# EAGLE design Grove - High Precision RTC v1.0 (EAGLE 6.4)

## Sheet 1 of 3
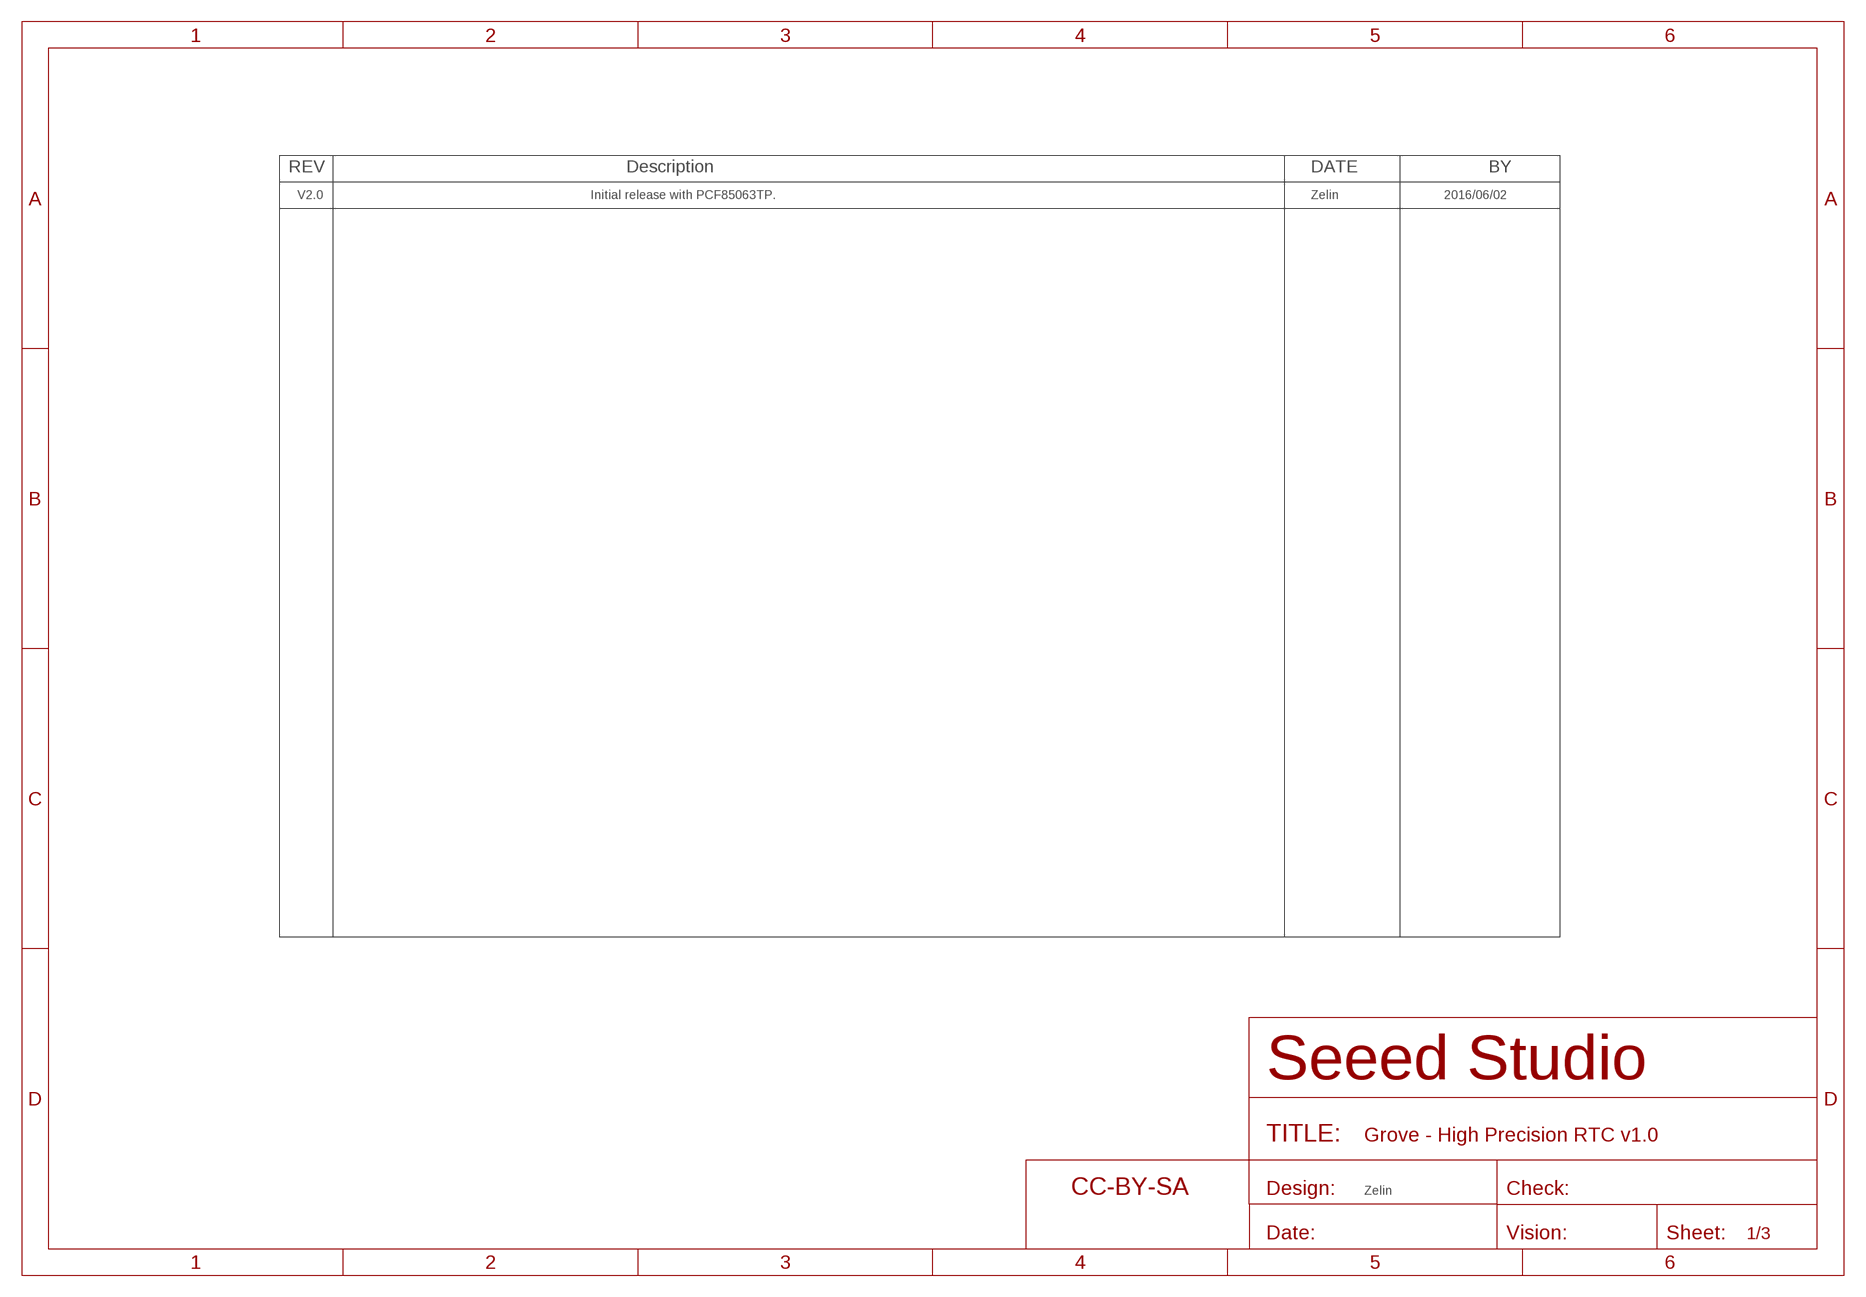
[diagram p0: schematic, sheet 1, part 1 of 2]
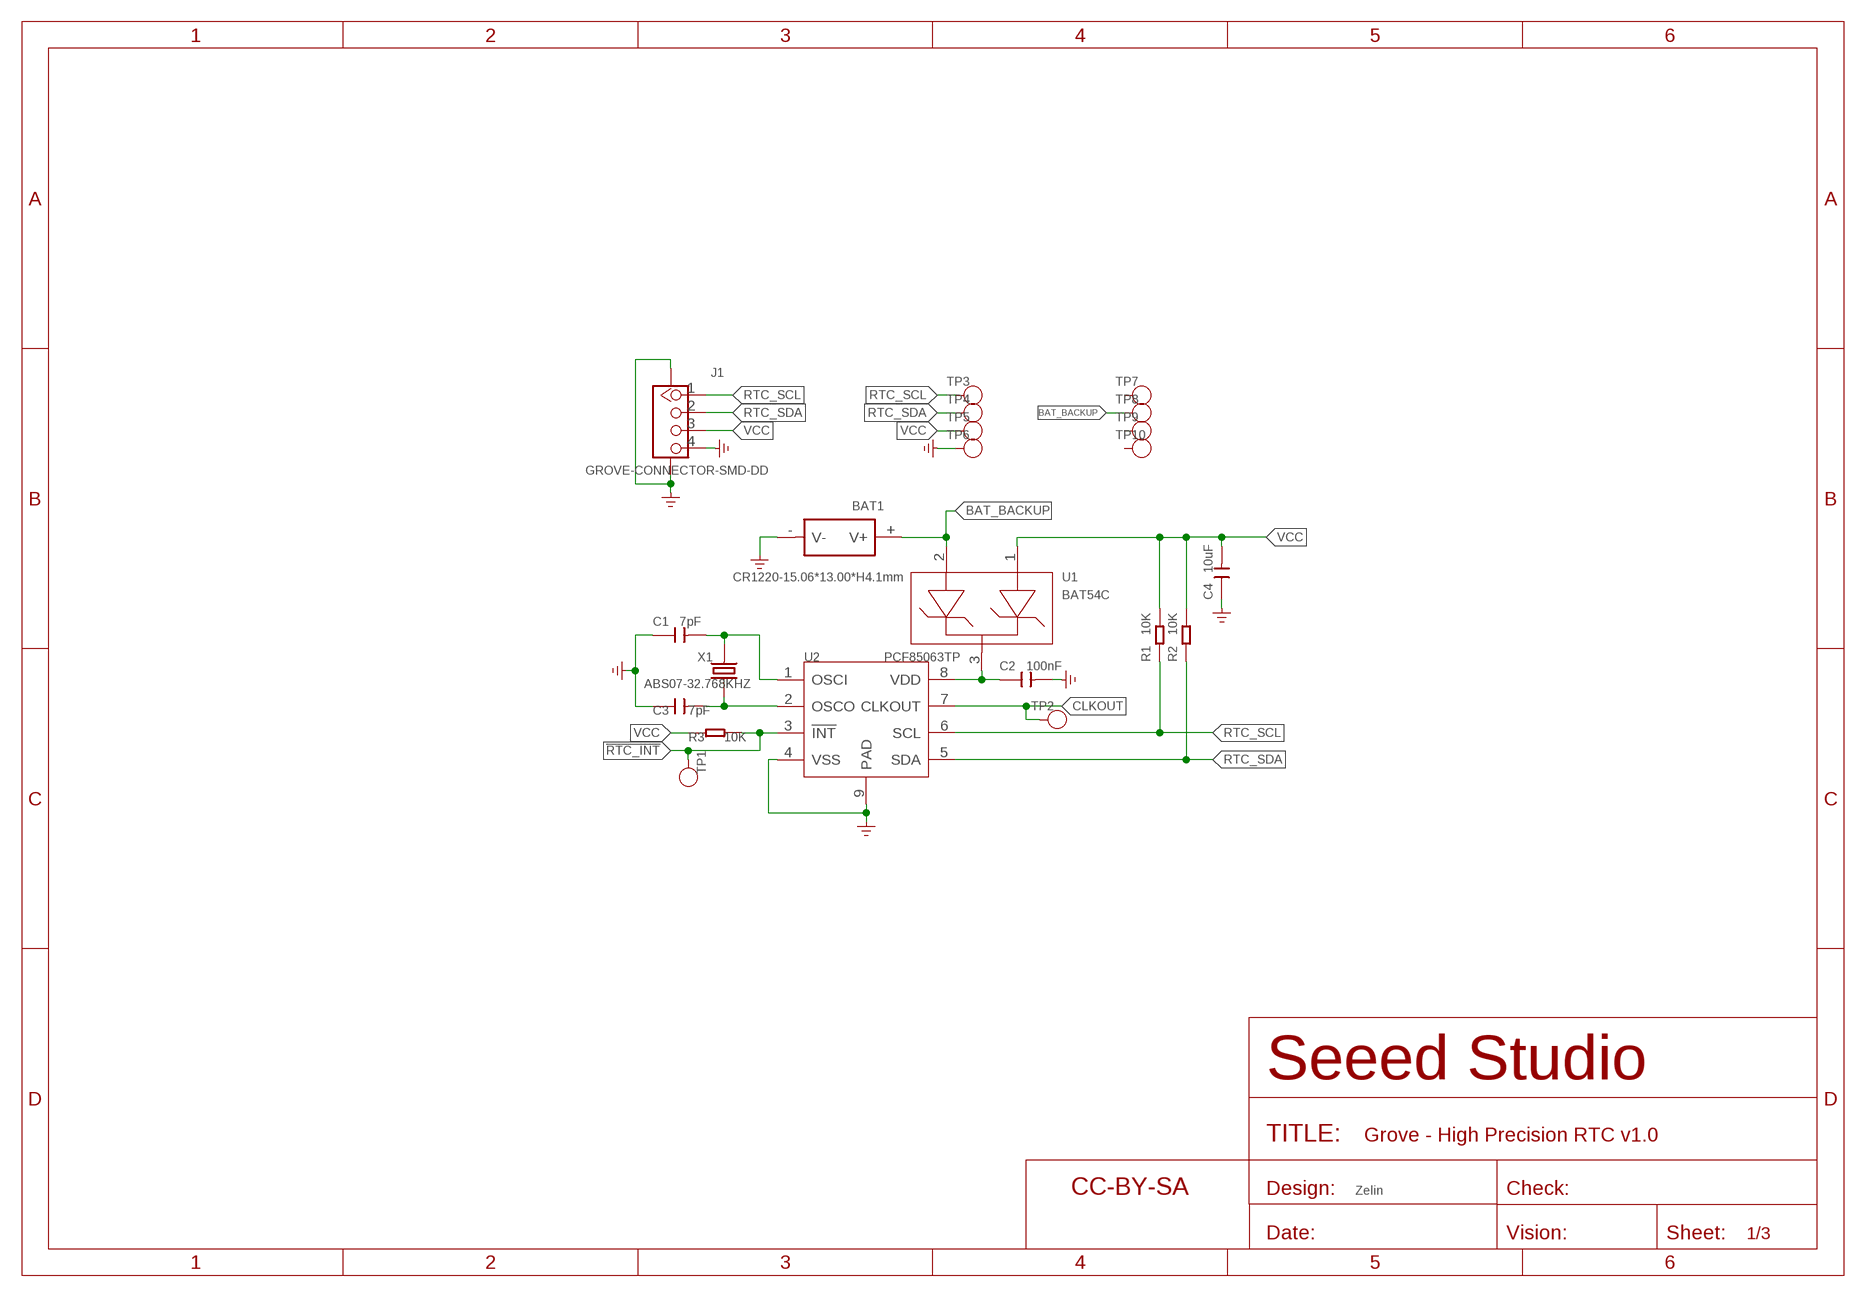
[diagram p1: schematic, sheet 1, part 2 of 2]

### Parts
BAT1  CR1220-15.06*13.00*H4.1mm  BAT-HOLDER'SMD-1220'  [BAT2P-SMD-16.4-CR1220]
C1  7pF  CAP-0402  [C0402]
C2  100nF  CAP-0402  [C0402]
C3  7pF  CAP-0402  [C0402]
C4  10uF  CAP-0805  [C0805]
FR  PG2  SEEEDSTUDIO-OPEN-SCH-FRAME  [SEEEDSTUDIO-PCB-FRAME]
FR1  PG1  SEEEDSTUDIO-OPEN-SCH-FRAME  [SEEEDSTUDIO-PCB-FRAME]
J1  GROVE-CONNECTOR-SMD-DD  GROVE-CONNECTOR-SMD'DD'  [HW4-SMD-2.0]
R1  10K  RES-0402  [R0402]
R2  10K  RES-0402  [R0402]
R3  10K  RES-0402  [R0402]
TP1  INT  TEST-POINT  [TP-D65/35MIL]
TP2  CLKOUT  TEST-POINT  [TP-D65/35MIL]
TP3  RTC_SCL  TEST-POINT'4545'  [TP-D45MIL]
TP4  RTC_SDA  TEST-POINT'4545'  [TP-D45MIL]
TP5  VCC  TEST-POINT'4545'  [TP-D45MIL]
TP6  GND  TEST-POINT'4545'  [TP-D45MIL]
TP7  RTC_SCL  TEST-POINT'4545'  [TP-D45MIL]
TP8  RTC_SDA  TEST-POINT'4545'  [TP-D45MIL]
TP9  VCC  TEST-POINT'4545'  [TP-D45MIL]
TP10  GND  TEST-POINT'4545'  [TP-D45MIL]
U1  BAT54C  DIODE-BAT54C  [SOT-23]
U2  PCF85063TP  RTC-PCF85063TP  [HWSON8-0.5-2X3X0.75MM]
X1  ABS07-32.768KHZ  CRYSTAL-2P-3215  [X2-SMD-3.2X1.5X0.55MM]

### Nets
!RTC_INT: R3.2 TP1.P1(T) U2.3(!INT)
BAT_BACKUP: BAT1.+(V+) TP8.T U1.2
CLKOUT: TP2.P1(T) U2.7(CLKOUT)
GND: BAT1.-(V-) C1.1 C2.2 C3.1 C4.1 J1.4 J1.SS1 J1.SS2 TP6.T U2.4(VSS) U2.9(PAD) ; supply symbol labelled GND_POWER
N$40: C3.2 U2.2(OSCO) X1.1
N$41: C1.2 U2.1(OSCI) X1.2
N$49: C2.1 U1.3 U2.8(VDD)
RTC_SCL: J1.1 R1.1 TP3.T U2.6(SCL)
RTC_SDA: J1.2 R2.1 TP4.T U2.5(SDA)
VCC: C4.2 J1.3 R1.2 R2.2 R3.1 TP5.T U1.1
Unconnected: TP7.T TP9.T TP10.T

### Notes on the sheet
- V2.0 | Initial release with PCF85063TP. | Zelin | 2016/06/02
- Zelin | Zelin

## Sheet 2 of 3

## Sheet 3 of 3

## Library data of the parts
BAT1 = Connector-new:BAT-HOLDER: BAT2P-13.5-CR1220:320170002;BAT2P-SMD-20.5-CR1632:320170007;METAL-CR2032-D20.0*H6.3MM:320170003;METAL-CR2032-SMD:320170006;PLASTIC-CR1220-L15.06*W13.0*H4.1MM:32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
C1-C4 = Discrete-new:CAP: Ceramic Capacitors
FR FR1 = moudle-new:SEEEDSTUDIO-OPEN-SCH-FRAME
J1 = Connector-new:GROVE-CONNECTOR-SMD: 4P-SMD-2.0:320110030;4P-SMD-2.0-90D:320110032
R1-R3 = Discrete-new:RES
TP1 TP2 = Discrete-new:TEST-POINT
TP3-TP10 = Discrete-new:TEST-POINT; PARTNO: DNP
U1 = Discrete-new:DIODE-BAT54C: Schottky barrier diodes
U2 = IC-new:RTC-PCF85063TP
X1 = Discrete-new:CRYSTAL-2P

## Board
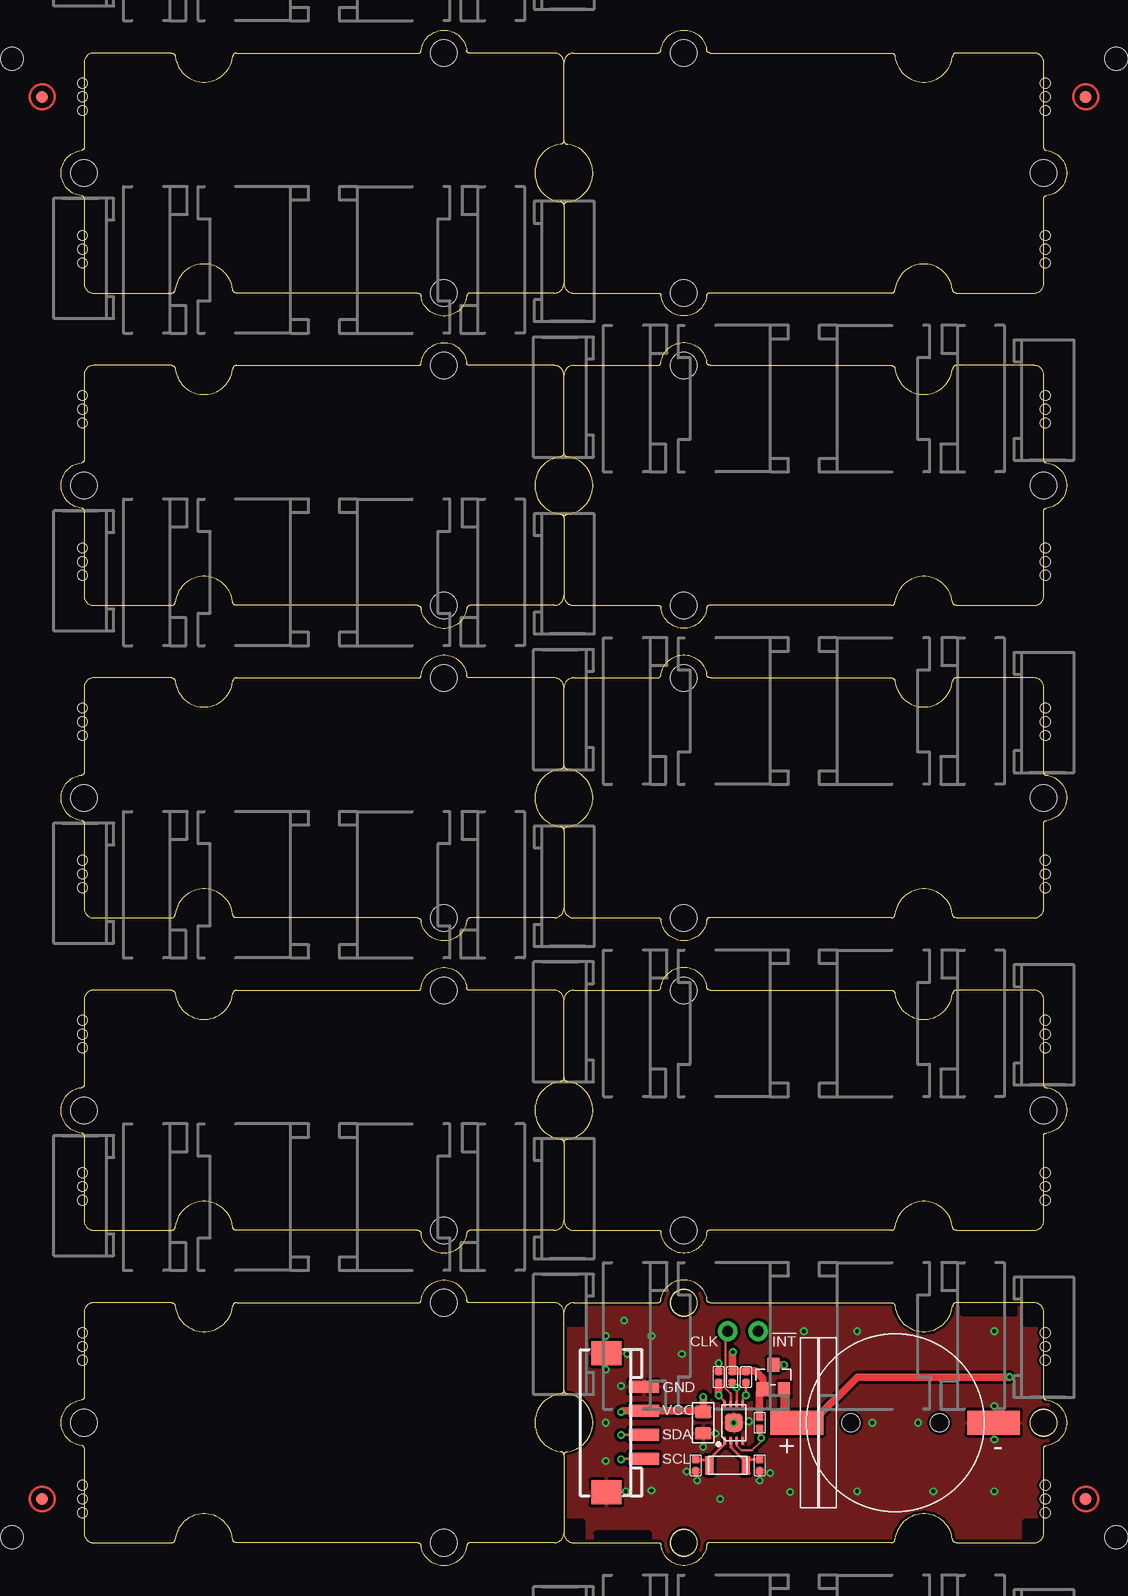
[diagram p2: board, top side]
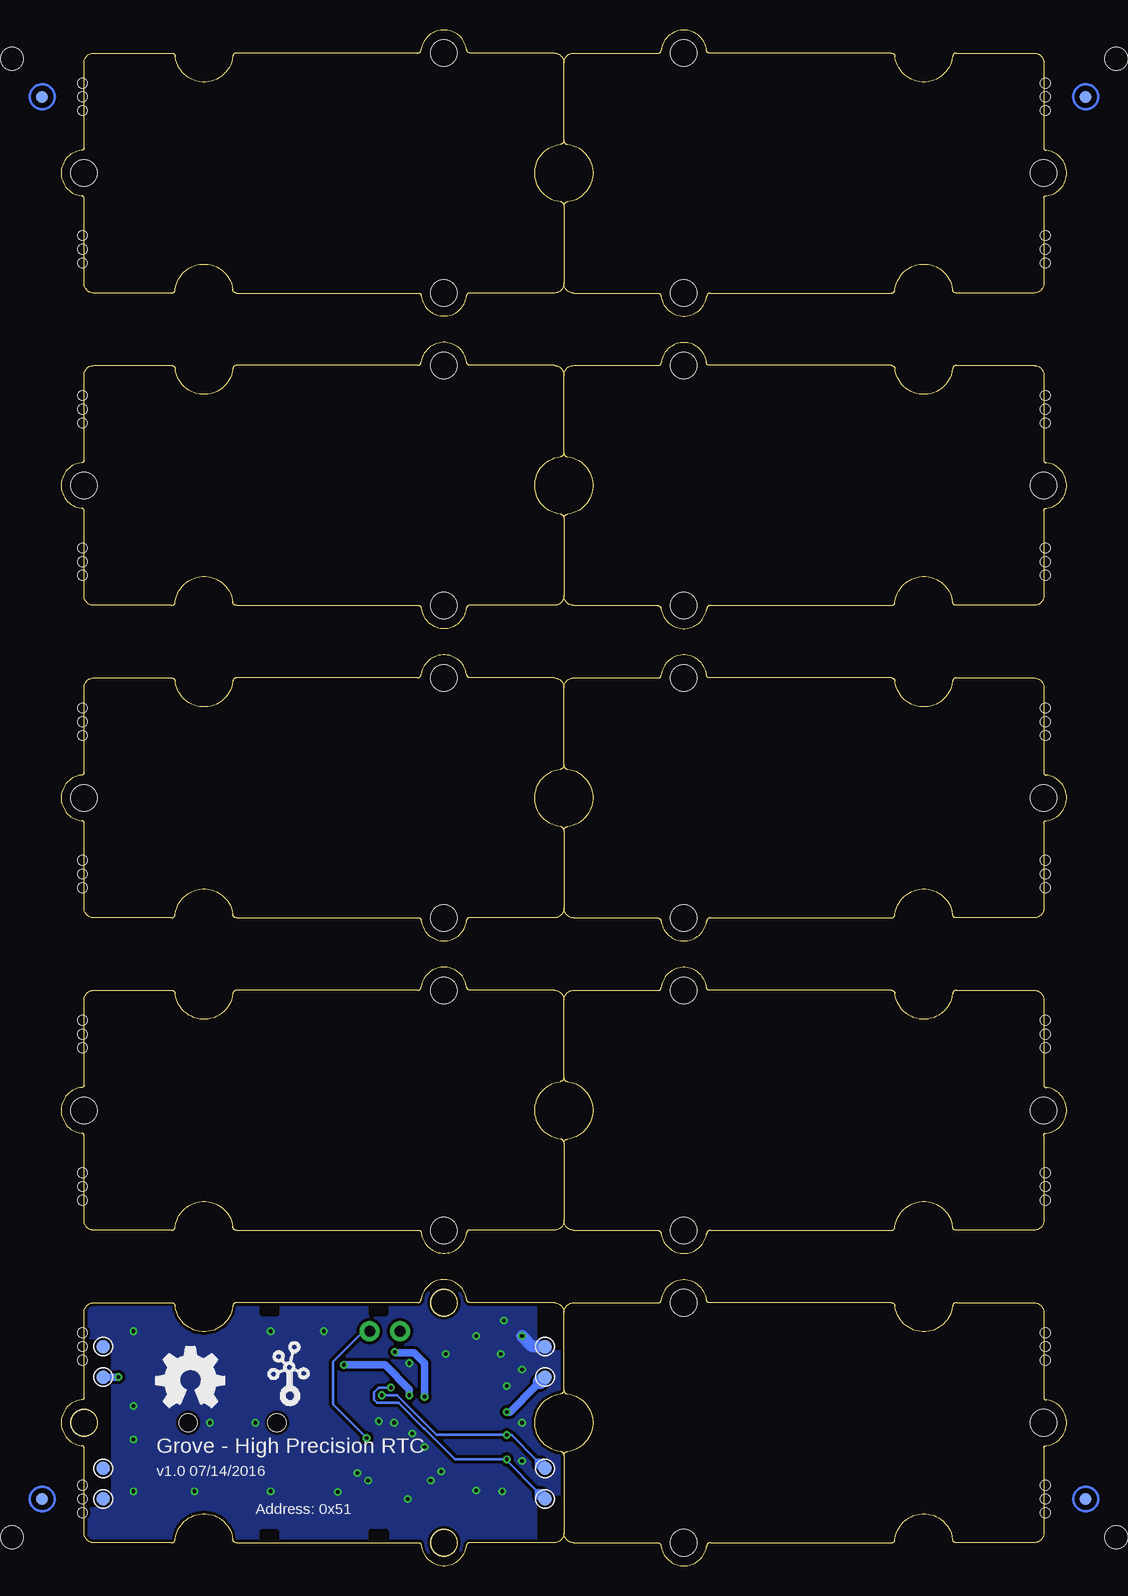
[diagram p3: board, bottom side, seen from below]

Size 83.82 x 127.98 mm. Coordinates in mm from the lower left corner, seen from the top.
Copper layers (1*16): Top 0.035mm / dielectric 1.5mm / Bottom 0.035mm
Design rules "SeeedStudio_2layer_DRU_no_angle_20140221 *": minimum track width 6mil, minimum drill 12mil, track to track 6mil, track to pad 6mil, pad to pad 6mil, via to via 6mil, smd to smd 0mil, copper to edge 10mil, drill to drill 10mil, minimum pad ring 10mil, minimum via ring 6mil, stop-mask expansion 2mil, vias tented up to drill 25mil, thermal gap 10mil
Holes 0.8 mm at 82.04,4.43 82.04,6.71 82.04,5.57 82.04,17.13 82.04,19.41 82.04,18.27 82.04,30.46 82.04,32.75 82.04,31.61 82.04,43.16 82.04,45.45 82.04,44.31 82.04,56.5 82.04,58.78 82.04,57.64 82.04,69.2 82.04,71.48 82.04,70.34 82.04,82.53 82.04,84.82 82.04,83.68 82.04,95.23 82.04,97.52 82.04,96.38 82.04,108.57 82.04,110.85 82.04,109.71 82.04,121.27 82.04,123.55 82.04,122.41 1.78,6.71 1.78,4.43 1.78,5.57 1.78,19.41 1.78,17.13 1.78,18.27 1.78,32.75 1.78,30.46 1.78,31.61 1.78,45.45 1.78,43.16 1.78,44.31 1.78,58.78 1.78,56.5 1.78,57.64 1.78,71.48 1.78,69.2 1.78,70.34 1.78,84.82 1.78,82.53 1.78,83.68 1.78,97.52 1.78,95.23 1.78,96.38 1.78,110.85 1.78,108.57 1.78,109.71 1.78,123.55 1.78,121.27 1.78,122.41
Holes 1.91 mm at 87.95,125.59 -4.13,125.59 -4.13,2.4 87.95,2.4

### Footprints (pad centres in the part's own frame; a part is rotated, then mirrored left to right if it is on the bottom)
BAT2P-SMD-16.4-CR1220 = smd 2 x 4.4: + 0,-8.2; - 0,8.2 | hole 1.5: 0,3.7; 0,-3.7
C0402 = smd 0.635 x 0.635: 1 0,0.484; 2 0,-0.484
C0805 = smd 1.397 x 1.016: 1 0,0.889; 2 0,-0.889
HW4-SMD-2.0 = smd 1 x 2.5: 1 -3,0; 2 -1,0; 3 1,0; 4 3,0 | smd 2 x 2.5: SS1 -5.8,3.123; SS2 5.8,3.123
ROUND-MARK-1.0 = smd 1.016 x 1.016: P$1 0,0
R0402 = smd 0.635 x 0.635: 1 0,0.484; 2 0,-0.484
TP-D65/35MIL = drill 0.889 pad 1.651: P1 0,0
TP-D45MIL = smd 1.143 x 1.143: T 0,0
SOT-23 = smd 1.016 x 1.143: 1 -0.889,-1.016; 2 0.889,-1.016; 3 0,1.016
HWSON8-0.5-2X3X0.75MM = smd 0.25 x 0.7: 1 -0.75,-1.5; 2 -0.25,-1.5; 3 0.25,-1.5; 4 0.75,-1.5; 5 0.75,1.5; 6 0.25,1.5; 7 -0.25,1.5; 8 -0.75,1.5 | smd 1.5 x 1.5: 9 0,0
GROVE-TEST-PLATFORM = hole 2.2: -10,-10; -10,10; 20,0
GROVE-1*2-TEST-PLATFORM-TOP = hole 2.2: 10.635,10; 10.635,-10; -19.365,0
X2-SMD-3.2X1.5X0.55MM = smd 0.762 x 1.524: 1 -1.524,0; 2 1.524,0

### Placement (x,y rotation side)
BAT1  69.53,11.92 270 top
C1  52.9,8.37 180 top
C2  54.8,15.73 180 top
C3  58.23,8.37 180 top
C4  53.53,11.92 180 top
FR  not placed on the board
FR1  not placed on the board
J1  48.58,11.92 90 top
P1  [ROUND-MARK-1.0]  85.41,122.41 180 top
P2  [ROUND-MARK-1.0]  -1.59,122.41 180 top
P3  [ROUND-MARK-1.0]  85.41,5.57 180 top
P4  [ROUND-MARK-1.0]  -1.59,5.57 180 top
P5  [ROUND-MARK-1.0]  85.41,122.41 180 bottom
P6  [ROUND-MARK-1.0]  -1.59,122.41 180 bottom
P7  [ROUND-MARK-1.0]  -1.59,5.57 180 bottom
P8  [ROUND-MARK-1.0]  85.41,5.57 180 bottom
R1  55.94,15.73 180 top
R2  57.09,15.73 180 top
R3  58.23,11.92 0 top
TP1  58.1,19.54 90 top
TP2  55.56,19.54 90 top
TP3  43.5,5.57 0 bottom
TP4  43.5,8.11 0 bottom
TP5  43.5,15.73 0 bottom
TP6  43.5,18.27 0 bottom
TP7  80.33,18.27 0 bottom
TP8  80.33,15.73 0 bottom
TP9  80.33,8.11 0 bottom
TP10  80.33,5.57 0 bottom
U1  59.37,15.73 0 top
U2  56.07,11.92 0 top
U3  [GROVE-TEST-PLATFORM]  21.91,90.03 180 top
U4  [GROVE-TEST-PLATFORM]  61.91,90.03 0 top
U5  [GROVE-TEST-PLATFORM]  21.91,63.99 180 top
U6  [GROVE-TEST-PLATFORM]  61.91,63.99 0 top
U7  [GROVE-TEST-PLATFORM]  21.91,37.96 180 top
U8  [GROVE-TEST-PLATFORM]  61.91,37.96 0 top
U11  [GROVE-TEST-PLATFORM]  21.91,11.92 180 top
U12  [GROVE-TEST-PLATFORM]  21.91,116.06 180 top
U13  [GROVE-TEST-PLATFORM]  61.91,116.06 0 top
U$5  [GROVE-1*2-TEST-PLATFORM-TOP]  62.55,11.92 180 top
U$16  [GROVE-SILK-SMALL]  66.99,13.19 0 bottom
U$17  [OSHW_FILLX200_NOTEXT]  75.88,13.19 0 bottom
X1  55.56,8.37 180 top

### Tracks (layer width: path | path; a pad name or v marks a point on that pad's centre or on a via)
!RTC_INT  (via drill 0.3 pad 0.64)
  Top 0.203: U2.3 56.32,10.02 56.71,9.64 57.6,9.64 58.36,10.4 v58.36,10.65 58.23,10.78 R3.2
  Bottom 0.203: TP1.P1 58.61,19.54 61.15,17 61.15,13.45 v58.36,10.65
BAT_BACKUP  (via drill 0.3 pad 0.64)
  Top 0.61: U1.2 60.26,12.56 60.9,11.92 BAT1.+ 62.55,11.92 66.36,15.73 v79.06,15.73
  Bottom 0.61: v79.06,15.73 TP8.T
CLKOUT
  Top 0.203: U2.7 55.82,14.33 55.37,14.78 55.37,19.35 TP2.P1
GND  (via drill 0.3 pad 0.64)
  Bottom 1.016: TP6.T 44.51,18.27 v45.4,19.16
  other vias: 46.67,14.97 54.8,16.87 45.4,16.37 45.4,11.92 47.05,6.21 53.02,7.1 66.36,6.21 77.79,6.21 77.79,10.52 77.79,13.32 61.91,19.54 66.36,19.54 77.79,19.54 53.53,9.89 52.13,7.86 58.23,7.1 45.4,8.75 47.18,17.64 51.75,17.64 59.12,7.73 56.07,11.92 57.34,12.05 54.55,11.03 72.71,6.21 49.21,19.16 49.21,6.27 71.44,11.92 67.63,11.92 46.93,20.43 60.77,6.14 54.93,5.57
  pour Top (isolate 0.254, rank 6): 40.96,22.72 82.23,22.72 82.23,1.13 40.96,1.13
  pour Bottom (isolate 0.254, rank 6): 40.96,22.72 82.23,22.72 82.23,1.13 40.96,1.13
N$40
  Top 0.254: U2.2 55.82,9.89 57.09,8.62 | X1.1 57.09,8.62 | C3.2 57.32,8.85 57.09,8.62
N$41
  Top 0.254: U2.1 55.32,10.16 54.04,8.87 54.04,8.75 | X1.2 54.04,8.75 | C1.2 53.94,8.85 54.04,8.75
N$49  (via drill 0.3 pad 0.64)
  Top 0.254: U2.8 55.32,13.69 v54.8,14.21
  Top 0.61: U1.3 v60.26,16.75 | C2.1 v54.8,14.21
  Bottom 0.61: v60.26,16.75 56.83,16.75 54.8,14.72 v54.8,14.21
RTC_SCL  (via drill 0.3 pad 0.64)
  Top 0.203: R1.1 55.94,15.22 v56.33,14.84 v56.32,14.84 U2.6 | J1.1 46.72,8.92 v46.67,8.87
  Bottom 0.203: 44.13,6.21 46.67,8.75 v46.67,8.87 50.99,8.87 53.53,11.41 53.59,11.48 55.69,13.57 57.47,13.57 57.72,13.83 57.72,14.46 57.34,14.84 v56.33,14.84 | 43.63,5.7 TP3.T
  Bottom 0.406: 44.13,6.21 43.63,5.7 | 44.13,6.21 43.75,6.21 43.37,5.83 | 44.13,6.21 44.13,5.83 43.75,5.44
RTC_SDA  (via drill 0.3 pad 0.64)
  Top 0.203: U2.5 56.82,13.94 v57.09,14.21 R2.1 | J1.2 46.69,10.92 v46.67,10.91
  Bottom 0.203: 44.13,8.75 46.29,10.91 v46.67,10.91 52.52,10.91 55.82,14.21 v57.09,14.21
  Bottom 0.406: 44.13,8.75 TP4.T | 44.13,8.75 43.75,8.75 43.24,8.24 | 44.13,8.75 44.13,8.37 43.75,7.98
VCC  (via drill 0.3 pad 0.64)
  Top 0.61: v46.67,12.81 46.78,12.92 J1.3 53.42,12.92 C4.2 v53.53,14.08 | v56.01,17.83 55.94,17.76 R1.2 R2.2 57.11,16.24 57.85,16.24 58.48,15.6 U1.1 58.23,14.46 R3.1
  Bottom 0.406: 43.24,15.48 43.75,14.97 44.26,14.97 44.26,15.48 43.88,15.86
  Bottom 0.61: v46.67,12.81 46.42,12.81 44.26,14.97 TP5.T | v53.53,14.08 53.53,16.87 54.42,17.76 55.94,17.76 v56.01,17.83

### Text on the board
tPlace: CLK | !INT | GND | VCC | SDA | SCL
bPlace: Grove - High Precision RTC | v1.0 07/14/2016 | Address: 0x51
tNames: + | -

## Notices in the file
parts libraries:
moudle-new: This work is licensed under the Creative Commons Attribution 4.0 International License.
To view a copy of this license,visit:
http://creativecommons.org/licenses/by-sa/4.0
moudle-new: CC-BY-SA
